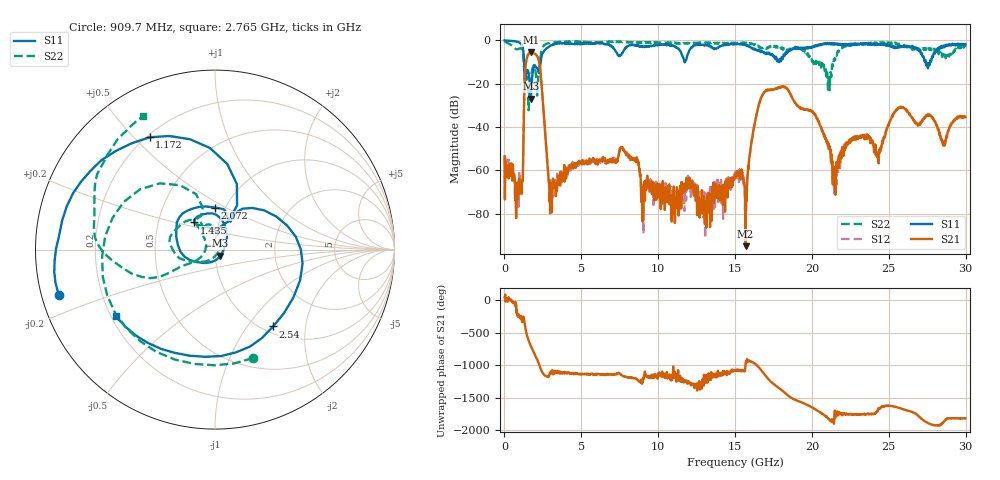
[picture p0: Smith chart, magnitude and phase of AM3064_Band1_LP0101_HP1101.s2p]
# Hz S DB R 50.0
!freq dBS11 angS11 dBS21 angS21 dBS12 angS12 dBS22 angS22
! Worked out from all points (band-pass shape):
!   1600 points, 10 MHz to 29.98 GHz, reference 50 ohm
!   highest |S21| = -5.47 dB at 1.716 GHz (marker M1); lowest = -95.0 dB at 15.68 GHz (marker M2)
!   |S21| within 3 dB of the highest: 1.445 GHz to 2.205 GHz (760 MHz wide, 41.7 % of centre)
!   lowest |S11| = -26.9 dB at 1.716 GHz (marker M3), VSWR 1.09, Z = 52.9 - j3.62 ohm
!   |S11| at or under -10 dB: 1.277 GHz to 2.355 GHz (1.078 GHz wide, 59.4 % of centre); 11.71061 GHz to 11.73563 GHz (25.01 MHz wide, 0.213 % of centre); 27.4 GHz to 27.68 GHz (282.6 MHz wide, 1.03 % of centre)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
!   |S22| runs from -32.2 to -0.4 dB; largest |S21 - S12| = 0.0077
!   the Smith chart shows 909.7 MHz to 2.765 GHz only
!   S11 on the Smith chart (normalised r, x): 909.7 MHz: 0.05, -0.14; 1.172 GHz: 0.21, +0.56; 1.435 GHz: 0.76, +0.24; 2.072 GHz: 0.90, +0.45; 2.54 GHz: 1.11, -1.34; 2.765 GHz: 0.22, -0.29
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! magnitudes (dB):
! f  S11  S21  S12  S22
! 10 MHz  0.0  -53.5  -53.7  -0.4
! 909.7 MHz  -0.8  -67.4  -67.4  -3.9
! 1.172 GHz  -2.8  -64.4  -65.5  -4.8
! 1.435 GHz  -14.4  -8.8  -8.7  -17.1
! 1.716 GHz  -26.9  -5.5  -5.5  -17.0
! 2.072 GHz  -12.6  -6.7  -6.6  -18.8
! 2.54 GHz  -5.4  -32.1  -32.1  -2.5
! 2.765 GHz  -3.5  -53.2  -54.9  -1.5
! 3.046 GHz  -2.2  -67.9  -70.0  -1.1
! 5.015 GHz  -1.5  -56.3  -56.1  -0.6
! 7.676 GHz  -5.6  -49.4  -49.5  -0.7
! 9.026 GHz  -2.9  -79.1  -73.5  -0.8
! 10 GHz  -2.0  -66.5  -72.3  -1.0
! 13.07 GHz  -1.9  -75.1  -81.8  -1.0
! 15 GHz  -1.7  -62.1  -61.9  -1.4
! 15.68 GHz  -2.2  -95.0  -69.5  -1.3
! 16.92 GHz  -5.7  -23.8  -23.6  -3.7
! 19.99 GHz  -3.4  -32.9  -32.7  -9.2
! 21.51 GHz  -1.4  -68.5  -65.4  -8.7
! 25 GHz  -2.0  -38.9  -38.3  -1.2
! 28.56 GHz  -2.7  -48.4  -48.7  -6.6
! 29.98 GHz  -1.7  -35.5  -35.2  -2.9
